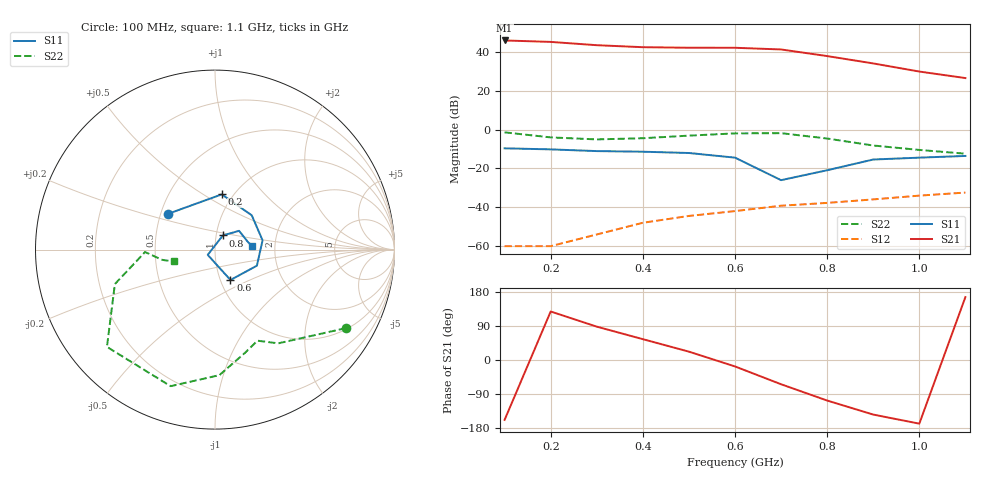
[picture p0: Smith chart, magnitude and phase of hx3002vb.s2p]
!  HPMX-3002  S PARAMETERS
!  Vcc1=4.5 V, Vcc2=6 V, Vcontrol = 2.0 V
!  LAST UPDATED 01 07 94
# ghz s ma r 50
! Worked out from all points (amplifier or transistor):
!   11 points, 100 MHz to 1.1 GHz, reference 50 ohm
!   highest |S21| = 45.9 dB at 100 MHz (marker M1)
!   |S21| within 3 dB of that: start of sweep to 354.3 MHz
!   unconditionally stable (mu >= 1): 111.7 MHz to 354.7 MHz; 957.1 MHz to end of sweep
!   at 200 MHz: K = 1.78, MAG = 47.5 dB, |S12| = -60.0 dB
!   at 600 MHz: K = 0.61, MSG = 42.0 dB, |S12| = -41.9 dB
!   at 1.1 GHz: K = 1.14, MAG = 27.2 dB, |S12| = -32.4 dB
!   S11 on the Smith chart (normalised r, x): 100 MHz: 0.54, +0.24; 200 MHz: 0.89, +0.60; 600 MHz: 1.12, -0.39; 800 MHz: 1.08, +0.17; 1.1 GHz: 1.53, +0.07
0.1  0.33 143.0  197.2 -158.0  0.001 153.0  0.85 -31.0
0.2  0.31 83.0  180.9 128.0  0.001 99.0  0.63 -56.0
0.3  0.28 43.0  148.9 88.0  0.002 142.0  0.56 -65.0
0.4  0.27 11.0  132.2 55.0  0.004 138.0  0.6 -74.0
0.5  0.25 -21.0  128.1 22.0  0.006 147.0  0.7 -88.0
0.6  0.19 -63.0  127.8 -17.0  0.008 143.0  0.8 -108.0
0.7  0.05 -144.0  115.6 -64.0  0.011 135.0  0.81 -138.0
0.8  0.09 61.0  78.15 -107.0  0.013 135.0  0.59 -161.0
0.9  0.17 38.0  50.54 -144.0  0.016 131.0  0.39 -178.0
1  0.19 12.0  31.23 -168.0  0.02 132.0  0.3 -169.0
1.1  0.21 6.0  21.22 166.0  0.024 127.0  0.24 -164.0
